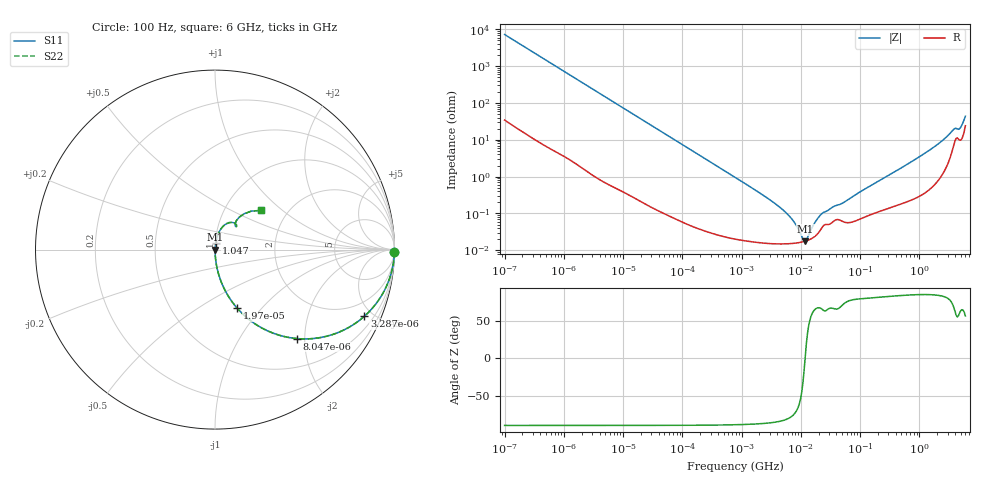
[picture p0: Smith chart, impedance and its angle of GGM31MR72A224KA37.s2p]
!Murata Part Number: GGM31MR72A224KA37
!These Parameters are Measured in Series Mode Connection
!Data Generated on Jun 19, 2026
!  o--ll--o
!Port1  Port2
!  o------o
!Operation Temp=25[degC], DC Bias Voltage=0[V]
!Freq. Start=100[Hz] Stop=6[GHz] 401[Steps]
# Hz S RI R 50
!Freq.(Hz) S11(Real) S11(Imag) S21(Real) S21(Imag) S12(Real) S12(Imag) S22(Real) S22(Imag)
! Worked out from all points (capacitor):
!   401 points, 100 Hz to 6 GHz, reference 50 ohm
!   read as one part in series: C = 219 nF near 109 Hz
!   lowest |Z| = 17.7 mohm at 11.89 MHz (marker M1)
!   series resonance near 11.81 MHz, so ESL is about 830 pH
!   S11 on the Smith chart (normalised r, x): 100 Hz: open; 3.287 kHz: 1.02, -4.46; 8.047 kHz: 1.01, -1.83; 19.7 kHz: 1.00, -0.75; 1.047 GHz: 1.01, +0.07; 6 GHz: 1.48, +0.73
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100  0.9997 -0.0138  0.000255 0.0138  0.000255 0.0138  0.9997 -0.0138
600  0.9929 -0.0816  0.00709 0.0816  0.00709 0.0816  0.9929 -0.0816
2008  0.9289 -0.2545  0.0711 0.2545  0.0711 0.2545  0.9289 -0.2545
3287  0.8315 -0.3721  0.1685 0.3721  0.1685 0.3721  0.8315 -0.3721
8047  0.4547 -0.4954  0.5453 0.4954  0.5453 0.4954  0.4547 -0.4954
19704  0.1241 -0.3269  0.8759 0.3269  0.8759 0.3269  0.1241 -0.3269
40335  0.0335 -0.1768  0.9665 0.1768  0.9665 0.1768  0.0335 -0.1768
129199  0.00376 -0.0572  0.9962 0.0572  0.9962 0.0572  0.00376 -0.0572
774597  0.000293 -0.0096  0.9997 0.0096  0.9997 0.0096  0.000293 -0.0096
5079039  0.00015 -0.00121  0.9998 0.00121  0.9998 0.00121  0.00015 -0.00121
7266822  0.000154 -0.000647  0.9998 0.000647  0.9998 0.000647  0.000154 -0.000647
1.087309e7  0.00017 -0.000107  0.9998 0.000107  0.9998 0.000107  0.00017 -0.000107
1.189169e7  0.000177 9.1e-06  0.9998 -9.1e-06  0.9998 -9.1e-06  0.000177 9.1e-06
1.300572e7  0.000185 0.000126  0.9998 -0.000126  0.9998 -0.000126  0.000185 0.000126
1.555665e7  0.000212 0.000366  0.9998 -0.000366  0.9998 -0.000366  0.000212 0.000366
2.327686e7  0.000433 0.00093  0.9996 -0.00093  0.9996 -0.00093  0.000433 0.00093
3.124326e8  0.00152 0.011  0.9985 -0.011  0.9985 -0.011  0.00152 0.011
1.046602e9  0.0043 0.0358  0.9957 -0.0358  0.9957 -0.0358  0.0043 0.0358
3.065283e9  0.0383 0.1222  0.9617 -0.1222  0.9617 -0.1222  0.0383 0.1222
3.8344e9  0.0939 0.152  0.9061 -0.152  0.9061 -0.152  0.0939 0.152
4.796499e9  0.1117 0.1416  0.8883 -0.1416  0.8883 -0.1416  0.1117 0.1416
6e9  0.2586 0.2184  0.7414 -0.2184  0.7414 -0.2184  0.2586 0.2184
